|   TEXAS INSTRUMENTS INCORPORATION
|   Package IBIS MODEL 144 GGU Package
[IBIS Ver]   2.1
[File Name]   sprm254.ibs
[File Rev]   1.0
[Date]   April 19, 2001
[Source]   IBIS Model Generated from PACED 4.40B
[Notes]
[Disclaimer]   Please be aware that in the absence of a written agreement
|   Texas Instruments(TI) assumes no liability for:
|   (1) The accuracy of the IBIS models provided to your company
|   (2) The proper functioning of these Models in your design
|   or for any resulting applications;or
|   (3)Infringement of patents,copyrights or intellectual
|   property rights resulting from your use of these models.
|   TI provides IBIS Models as a service to our customers and
|   therefore reserves the right to limit distribution of the
|   Models.
[Copyright]   Property of Texas Instruments Incorporated.
|   Unauthorised reproduction and/or distribution is strictly
|   prohibited.
|   This product is protected under copyright law and trade
|   secret law as an unpublished work.
|   Created 1999,(C) Copyright 1999-2001,
|   Texas Instruments Incorporated., All Rights Reserved.
|   These commodities are under the U.S.
|   Government distribution license control.As such,they are not
|   to be re-exported without the prior approval of the U.S.
|   Department of Commerce.
[component]   F741588
[Manufacturer]   Texas Instruments Inc.
[Package]
| variable   typ   min   max
R_pkg   9.149711e-002  3.193799e-002  1.737291e-001
L_pkg   2.553001e-009  1.081282e-009  4.775501e-009
C_pkg   2.167484e-013  1.789633e-013  2.766307e-013
[Pin] signal_name  model_name   R_pin   L_pin   C_pin
1   GND   GND   1.4093E-01   4.0808E-09   2.5376E-13
2   PA22   OUK831/UPS239   1.3096E-01   3.5036E-09   2.3065E-13
3   GND   GND   8.9196E-02   2.5352E-09   2.4121E-13
4   POWER   POWER   1.1988E-01   3.2399E-09   2.1719E-13
5   A10   OUK831/UPS239   6.8051E-02   1.9424E-09   2.5215E-13
6   HD7   OUK831/UPS239   8.8648E-02   2.3739E-09   2.0974E-13
7   A11   OUK831/UPS239   8.2067E-02   2.3623E-09   2.1987E-13
8   A12   OUK831/UPS239   1.0984E-01   3.0356E-09   2.2313E-13
9   A13   OUK831/UPS239   4.4149E-02   1.2957E-09   2.0548E-13
10   A14   OUK831/UPS239   8.2763E-02   2.2542E-09   1.9902E-13
11   A15   OUK831/UPS239   7.8188E-02   2.2582E-09   2.0331E-13
12   POWER   POWER   8.0150E-02   2.8499E-09   2.5386E-13
13   HAS_   IDG091_PS1001   1.6183E-01   4.3998E-09   2.5235E-13
14   GND   GND   7.2146E-02   1.9497E-09   1.8989E-13
15   GND   GND   7.9268E-02   2.2181E-09   1.9631E-13
16   POWER   POWER   7.6708E-02   2.7176E-09   2.2291E-13
17   HCS_   IDG091_PS1001   1.1013E-01   2.9889E-09   2.4272E-13
18   HRW   IDG041_PS1001   1.0778E-01   2.8026E-09   2.1961E-13
19   READY   IDG041   1.4320E-01   3.9004E-09   2.5369E-13
20   PS_   OUK831   9.9085E-02   2.7441E-09   2.2162E-13
21   DS_   OUK831   9.2703E-02   2.6840E-09   1.8355E-13
22   IS_   OUK831   7.6415E-02   2.0546E-09   1.8650E-13
23   RW_   OUK831   4.4818E-02   1.2700E-09   1.7899E-13
24   MSTRB_   OUK831   1.1462E-01   3.0331E-09   2.3481E-13
25   IOSTRB_   OUK831   9.6732E-02   2.8513E-09   2.1991E-13
26   MSC_   OUK831   8.1214E-02   2.1047E-09   2.0855E-13
27   XF   OUK831   4.3791E-02   1.3761E-09   2.0221E-13
28   HOLDA_   OUK831   4.2172E-02   1.2234E-09   2.0480E-13
29   IAQ_   OUK831   1.1123E-01   3.0425E-09   2.1993E-13
30   HOLD_   IDG041   8.8372E-02   2.3338E-09   2.1197E-13
31   BIO_   IDG091   5.1369E-02   1.5727E-09   2.0793E-13
32   MPNMC_   IDG041   1.1691E-01   3.2732E-09   2.3286E-13
33   POWER   POWER   9.4959E-02   2.6177E-09   2.1290E-13
34   GND   GND   7.8757E-02   2.1622E-09   2.4351E-13
35   BDR1   IDG041   1.2816E-01   3.5910E-09   2.4946E-13
36   BFSR1   OUK831/IDG041   1.0322E-01   2.8207E-09   2.0217E-13
37   GND   GND   1.4175E-01   4.0687E-09   2.4731E-13
38   BCLKR1   OUK831/IDG091   1.3098E-01   3.5129E-09   2.1993E-13
39   HCNTL0   IDG041_PS1001   9.5280E-02   2.6647E-09   2.3027E-13
40   GND   GND   1.1868E-01   3.2119E-09   2.0602E-13
41   BCLKR0   OUK831/IDG091   6.6053E-02   1.8990E-09   2.4667E-13
42   BCLKR2   OUK831/IDG091   8.7037E-02   2.3323E-09   2.0755E-13
43   BFSR0   OUK831/IDG041   8.3931E-02   2.3596E-09   1.9873E-13
44   BFSR2   OUK831/IDG041   1.0758E-01   2.9843E-09   2.1457E-13
45   BDR0   IDG041   4.0710E-02   1.2112E-09   2.0515E-13
46   HCNTL1   IDG041_PS1001   8.1398E-02   2.2242E-09   1.9826E-13
47   BDR2   IDG041   7.6325E-02   2.2163E-09   2.0185E-13
48   BCLKX0   OUK831/IDG091   1.0636E-01   2.9515E-09   2.1736E-13
49   BCLKX2   OUK831/IDG091   3.7688E-02   1.1159E-09   1.8665E-13
50   GND   GND   6.8400E-02   1.8721E-09   1.8601E-13
51   HINT   OUK831   7.1479E-02   2.0842E-09   2.0427E-13
52   POWER   POWER   9.7153E-02   2.6869E-09   1.8589E-13
53   BFSX0   OUK831/IDG041   6.9972E-02   2.0515E-09   1.8076E-13
54   BFSX2   OUK831/IDG041   1.0967E-01   3.0873E-09   1.8950E-13
55   HRDY   OUK831   4.0321E-02   1.1141E-09   2.0625E-13
56   POWER   POWER   9.4143E-02   2.6468E-09   2.1675E-13
57   GND   GND   8.8995E-02   2.5947E-09   1.7896E-13
58   HD0   OUK831/UPS239   7.2958E-02   1.9769E-09   1.8394E-13
59   BDX0   OUK831   4.1165E-02   1.1804E-09   1.8097E-13
60   BDX2   OUK831   1.0967E-01   2.9528E-09   2.3252E-13
61   IACK_   OUK831   9.4254E-02   2.7890E-09   2.1791E-13
62   HBIL   IDG041_PS1001   7.8017E-02   2.0272E-09   2.0570E-13
63   NMI_   IDG091   4.0727E-02   1.2949E-09   2.0513E-13
64   INT0_   IDG091   4.1807E-02   1.2688E-09   2.0332E-13
65   INT1_   IDG091   1.0916E-01   2.9957E-09   2.1851E-13
66   INT2_   IDG091   8.6818E-02   2.2756E-09   2.1356E-13
67   INT3_   IDG091   4.9996E-02   1.5625E-09   2.0512E-13
68   POWER   POWER   1.1581E-01   3.2195E-09   2.3152E-13
69   HD1   OUK831/UPS239   9.4127E-02   2.6007E-09   2.1176E-13
70   GND   GND   7.8934E-02   2.1548E-09   2.4247E-13
71   BCLKX1   OUK831/IDG091   1.2778E-01   3.5819E-09   2.4931E-13
72   GND   GND   1.0179E-01   2.7503E-09   2.1132E-13
73   BFSX1   OUK831/IDG041   1.4083E-01   4.0785E-09   2.5360E-13
74   BDX1   OUK831   1.3117E-01   3.5087E-09   2.3081E-13
75   POWER   POWER   8.9378E-02   2.5396E-09   2.4140E-13
76   GND   GND   1.2005E-01   3.2443E-09   2.1716E-13
77   CLKMD1   IDG091   6.8201E-02   1.9460E-09   2.5229E-13
78   CLKMD2   IDG091   8.8559E-02   2.3718E-09   2.0977E-13
79   CLKMD3   IDG091   8.1719E-02   2.3538E-09   2.1959E-13
80   HPI16   IDG041_PE1001   1.0930E-01   3.0227E-09   2.2281E-13
81   HD2   OUK831/UPS239   4.3462E-02   1.2791E-09   2.0452E-13
82   TOUT   OUK831   8.2012E-02   2.2361E-09   1.9798E-13
83   EMU0   OUK831/IDG041   7.7791E-02   2.2535E-09   2.0247E-13
84   EMU1   OUK831/IDG041   1.0877E-01   3.0149E-09   2.2178E-13
85   TDO   OUK831   4.0970E-02   1.1957E-09   1.9202E-13
86   TDI   IDG041_PS1001   7.1975E-02   1.9458E-09   1.8973E-13
87   TRST_   IDG041_PE1001   7.9126E-02   2.2147E-09   1.9616E-13
88   TCK   IDG091_PS1001   1.0109E-01   2.7811E-09   1.9107E-13
89   TMS   IDG041_PS1001   7.3431E-02   2.1385E-09   1.8778E-13
90   GND   GND   1.1367E-01   3.1829E-09   1.9118E-13
91   POWER   POWER   3.1938E-02   1.1876E-09   1.9940E-13
92   HPIENA   IDG041_PE1001   9.9195E-02   2.7467E-09   2.2170E-13
93   GND   GND   9.2867E-02   2.6875E-09   1.8368E-13
94   CLKOUT   OUKB31   7.6645E-02   2.0604E-09   1.8652E-13
95   HD3   OUK831/UPS239   4.4901E-02   1.2715E-09   1.7963E-13
96   X1   NC   1.1458E-01   3.0413E-09   2.3529E-13
97   X2CLKIN   UIS434   9.7304E-02   2.8650E-09   2.2030E-13
98   RS_   IDG041   8.2023E-02   2.1240E-09   2.0923E-13
99   D0   OUK831/UPS239   4.4779E-02   1.4001E-09   2.0310E-13
100   D1   OUK831/UPS239   4.3415E-02   1.2534E-09   2.0581E-13
101   D2   OUK831/UPS239   1.1255E-01   3.0743E-09   2.2116E-13
102   D3   OUK831/UPS239   8.9731E-02   2.3667E-09   2.1317E-13
103   D4   OUK831/UPS239   5.2457E-02   1.5991E-09   2.0883E-13
104   D5   OUK831/UPS239   1.1784E-01   3.2959E-09   2.3393E-13
105   PA16   OUK831/UPS239   9.5730E-02   2.6367E-09   2.1368E-13
106   GND   GND   7.9165E-02   2.1723E-09   2.4418E-13
107   PA17   OUK831   1.2861E-01   3.6019E-09   2.4987E-13
108   PA18   OUK831   1.0356E-01   2.8229E-09   2.0205E-13
109   PA19   OUK831   1.4200E-01   4.0788E-09   2.4736E-13
110   PA20   OUK831   1.3111E-01   3.5163E-09   2.2006E-13
111   GND   GND   9.5365E-02   2.6667E-09   2.3008E-13
112   POWER   POWER   1.1881E-01   3.2153E-09   2.0616E-13
113   D6   OUK831/UPS239   6.6163E-02   1.9020E-09   2.4681E-13
114   D7   OUK831/UPS239   8.7120E-02   2.3349E-09   2.0760E-13
115   D8   OUK831/UPS239   8.4051E-02   2.3632E-09   1.9917E-13
116   D9   OUK831/UPS239   1.0776E-01   2.9879E-09   2.1488E-13
117   D10   OUK831/UPS239   4.0880E-02   1.2148E-09   2.0518E-13
118   D11   OUK831/UPS239   7.9738E-02   2.1842E-09   1.9682E-13
119   D12   OUK831/UPS239   7.4802E-02   2.1799E-09   2.0052E-13
120   HD4   OUK831/UPS239   1.0512E-01   2.9202E-09   2.1704E-13
121   D13   OUK831/UPS239   3.6227E-02   1.0813E-09   1.8519E-13
122   D14   OUK831/UPS239   6.7771E-02   1.8499E-09   1.8511E-13
123   D15   OUK831/UPS239   7.0853E-02   2.0705E-09   2.0364E-13
124   HD5   OUK831/UPS239   9.6815E-02   2.6792E-09   1.8556E-13
125   POWER   POWER   7.5090E-02   2.7632E-09   2.3987E-13
126   GND   GND   1.0385E-01   2.7048E-09   2.1727E-13
127   HDS1   IDG091_PS1001   1.3831E-01   3.7859E-09   2.6276E-13
128   GND   GND   9.4326E-02   2.6513E-09   2.1689E-13
129   HDS2   IDG091_PS1001   8.9164E-02   2.5985E-09   1.7910E-13
130   POWER   POWER   7.3122E-02   1.9806E-09   1.8410E-13
131   A0   OUK831/UPS239   4.1359E-02   1.1852E-09   1.8112E-13
132   A1   OUK831/UPS239   1.6845E-01   4.5461E-09   2.6316E-13
133   A2   OUK831/UPS239   1.1015E-01   2.8775E-09   2.7663E-13
134   A3   OUK831/UPS239   1.0931E-01   2.9231E-09   2.3247E-13
135   HD6   OUK831/UPS239   1.4241E-01   3.8293E-09   2.6801E-13
136   A4   OUK831/UPS239   1.7373E-01   4.7755E-09   2.6640E-13
137   A5   OUK831/UPS239   1.1683E-01   2.9756E-09   2.4884E-13
138   A6   OUK831/UPS239   1.2041E-01   3.2260E-09   2.4171E-13
139   A7   OUK831/UPS239   1.4913E-01   3.9578E-09   2.6838E-13
140   A8   OUK831/UPS239   1.2493E-01   3.2809E-09   2.6045E-13
141   A9   OUK831/UPS239   1.3049E-01   3.3867E-09   2.4428E-13
142   POWER   POWER   6.4070E-02   2.1024E-09   2.4413E-13
143   PA21   OUK831   1.2785E-01   3.5837E-09   2.4971E-13
144   GND   GND   1.0189E-01   2.7532E-09   2.1137E-13
[Component]   UIS434
[Manufacturer]   Texas Instruments
[Package]
|   typ   min   max
R_pkg   0   0   0
L_pkg   0   0   0
C_pkg   0   0   0
[Pin]   signal_name   model_name   R_pin   L_pin   C_pin
   1   XI   UIS434   0   0   0
[Component]   IDG091
[Manufacturer]   Texas Instruments
[Package]
|   typ   min   max
R_pkg   0   0   0
L_pkg   0   0   0
C_pkg   0   0   0
[Pin]   signal_name   model_name   R_pin   L_pin   C_pin
   1   A   IDG091   0   0   0
[Component]   IDG041_PE1001
[Manufacturer]   Texas Instruments
[Package]
|   typ   min   max
R_pkg   0   0   0
L_pkg   0   0   0
C_pkg   0   0   0
[Pin]   signal_name   model_name   R_pin   L_pin   C_pin
   1   A   IDG041_PE1001   0   0   0
[Component]   IDG041
[Manufacturer]   Texas Instruments
[Package]
|   typ   min   max
R_pkg   0   0   0
L_pkg   0   0   0
C_pkg   0   0   0
[Pin]   signal_name   model_name   R_pin   L_pin   C_pin
   1   A   IDG041   0   0   0
[Component]   IDG041_PS1001
[Manufacturer]   Texas Instruments
[Package]
|   typ   min   max
R_pkg   0   0   0
L_pkg   0   0   0
C_pkg   0   0   0
[Pin]   signal_name   model_name   R_pin   L_pin   C_pin
   1   A   IDG041_PS1001   0   0   0
[Component]   IDG091_PS1001
[Manufacturer]   Texas Instruments
[Package]
|   typ   min   max
R_pkg   0   0   0
L_pkg   0   0   0
C_pkg   0   0   0
[Pin]   signal_name   model_name   R_pin   L_pin   C_pin
   1   A   IDG091_PS1001   0   0   0
[Component]   OUK831
[Manufacturer]   Texas Instruments
[Package]
|   typ   min   max
R_pkg   0   0   0
L_pkg   0   0   0
C_pkg   0   0   0
[Pin]   signal_name   model_name   R_pin   L_pin   C_pin
   1   Y   OUK831   0   0   0
[Component]   OUKB31
[Manufacturer]   Texas Instruments
[Package]
|   typ   min   max
R_pkg   0   0   0
L_pkg   0   0   0
C_pkg   0   0   0
[Pin]   signal_name   model_name   R_pin   L_pin   C_pin
   1   Y   OUKB31   0   0   0
[Component]   UPS239
[Manufacturer]   Texas Instruments
[Package]
|   typ   min   max
R_pkg   0   0   0
L_pkg   0   0   0
C_pkg   0   0   0
[Pin]   signal_name   model_name   R_pin   L_pin   C_pin
   1   A   UPS239   0   0   0
| Models and submodels in the file (9): UIS434 (Input), IDG091 (Input), IDG041_PE1001 (Input), IDG041 (Input), IDG041_PS1001 (Input), IDG091_PS1001 (Input), OUK831 (3-state), OUKB31 (3-state), UPS239 (Input)
